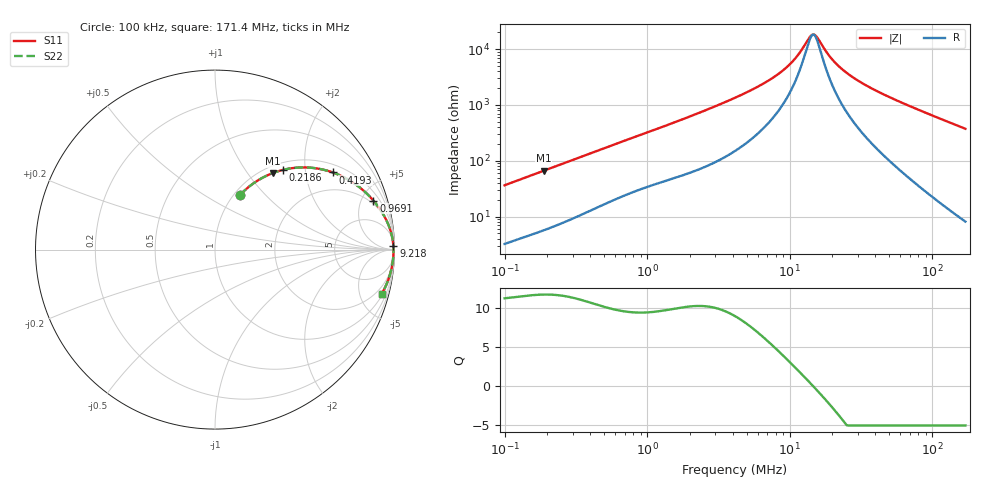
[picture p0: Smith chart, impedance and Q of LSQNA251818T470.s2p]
! LSQNA251818T470  S-PARAMETER MODEL  ( General Type )
! Model Generated by TAIYO YUDEN Corporation (http://www.ty-top.com)
! Version 2.0
! TAIYO YUDEN Control No. 100810NF25SB-FKC
! Copyright(c) 2007 TAIYO YUDEN CO.,LTD. All Rights Reserved.
! Product Description (link to TY-COMPAS)
! https://ds.yuden.co.jp/TYCOMPAS/or/detail?pn=LSQNA251818T470K&u=M
! Products Name : Inductors
! Characteristics :
!  Inductance : 47 uH , SRF(min) : 12 MHz , DC Resistance(max) : 1.235 Ohm
!  Rated Current : Saturation :110 mA , Temp Rise : 420 mA (40 degC)
!  Case Size : 2.5 x 1.8 / 0.098 x 0.071 [mm/inch] , Thickness : 1.8 / 0.071 [mm/inch]
!  (Conditions: Temperature = 25 degC , DC Bias Current/Voltage = 0A / 0V)
! External Node Assignments :
!  1  o---GGG---o  2
! GND o---------o GND
! Frequency Range : 0.1MHz  -  171.398534MHz  [ 402 STEP ]
# MHz S RI R 50
! Freq[MHz].  S11 Real  S11 Imag  S21 Real  S21 Imag  S12 Real  S12 Imag  S22 Real  S22 Imag
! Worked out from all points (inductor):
!   401 points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, 100 kHz to 171.4 MHz, reference 50 ohm
!   read as one part in series: L = 57 uH near 103.8 kHz
!   highest Q = 11.7 at 188.3 kHz (marker M1), where L = 56 uH
!   self-resonance near 14.41 MHz
!   S11 on the Smith chart (normalised r, x): 100 kHz: 1.06, +0.72; 218.6 kHz: 1.13, +1.53; 419.3 kHz: 1.27, +2.84; 969.1 kHz: 1.66, +6.20; 9.218 MHz: 24, +85; 171.4 MHz: 1.16, -7.48
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0.1  0.1376 0.3028  0.8624 -0.3028  0.8624 -0.3028  0.1376 0.3028
0.188317  0.3209 0.426  0.6791 -0.426  0.6791 -0.426  0.3209 0.426
0.21856  0.3805 0.4445  0.6195 -0.4445  0.6195 -0.4445  0.3805 0.4445
0.348094  0.5818 0.4498  0.4182 -0.4498  0.4182 -0.4498  0.5818 0.4498
0.419321  0.6571 0.4296  0.3429 -0.4296  0.3429 -0.4296  0.6571 0.4296
0.631563  0.7912 0.358  0.2088 -0.358  0.2088 -0.358  0.7912 0.358
0.969108  0.883 0.2726  0.117 -0.2726  0.117 -0.2726  0.883 0.2726
1.211692  0.9154 0.2309  0.0846 -0.2309  0.0846 -0.2309  0.9154 0.2309
2.324706  0.969 0.1313  0.031 -0.1313  0.031 -0.1313  0.969 0.1313
4.140031  0.9865 0.0723  0.0135 -0.0723  0.0135 -0.0723  0.9865 0.0723
6.593697  0.9919 0.0399  0.0081 -0.0399  0.0081 -0.0399  0.9919 0.0399
9.21848  0.9937 0.0217  0.00635 -0.0217  0.00635 -0.0217  0.9937 0.0217
11.10477  0.9942 0.0128  0.00581 -0.0128  0.00581 -0.0128  0.9942 0.0128
13.62839  0.9945 0.00331  0.00549 -0.00331  0.00549 -0.00331  0.9945 0.00331
14.41119  0.9946 0.000773  0.00544 -0.000773  0.00544 -0.000773  0.9946 0.000773
15.52529  0.9946 -0.00261  0.0054 0.00261  0.0054 0.00261  0.9946 -0.00261
19.41154  0.9945 -0.0129  0.00546 0.0129  0.00546 0.0129  0.9945 -0.0129
24.27059  0.9942 -0.0239  0.00581 0.0239  0.00581 0.0239  0.9942 -0.0239
32.69193  0.9932 -0.0405  0.00684 0.0405  0.00684 0.0405  0.9932 -0.0405
50.16444  0.9897 -0.0709  0.0103 0.0709  0.0103 0.0709  0.9897 -0.0709
94.4684  0.9745 -0.1403  0.0255 0.1403  0.0255 0.1403  0.9745 -0.1403
171.3985  0.9287 -0.2467  0.0713 0.2467  0.0713 0.2467  0.9287 -0.2467
